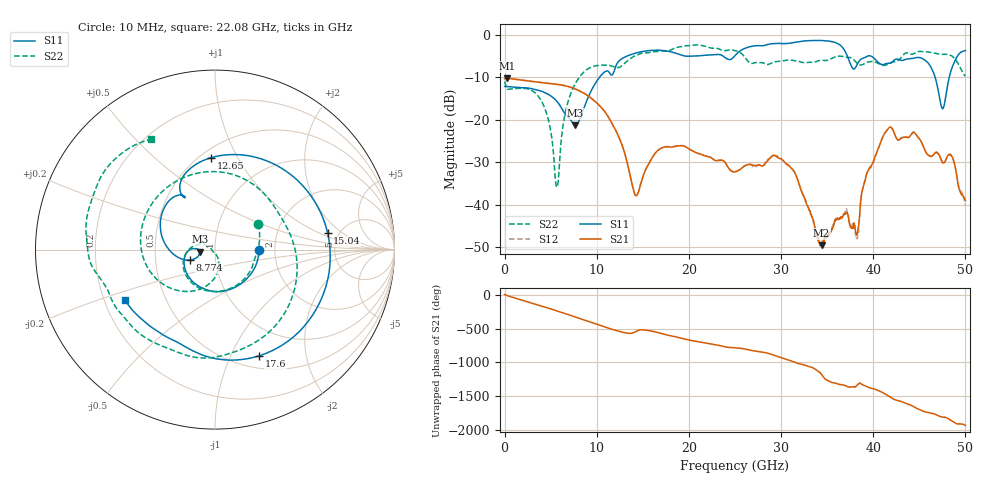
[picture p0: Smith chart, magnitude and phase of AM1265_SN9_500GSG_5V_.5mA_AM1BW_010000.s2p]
!Keysight Technologies,N5245B,MY58422270,A.16.20.02
!Date: Thursday, March 05, 2026 00:52:19
!Correction: S11(C  2-Port  )
!S21(C  2-Port  )
!S12(C  2-Port  )
!S22(C  2-Port  )
!S2P File: Measurements: S11, S21, S12, S22:
# Hz S  dB  R 50
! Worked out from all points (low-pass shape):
!   3201 points, 10 MHz to 50 GHz, reference 50 ohm
!   highest |S21| = -10.31 dB at 275.6 MHz (marker M1); lowest = -49.5 dB at 34.39 GHz (marker M2)
!   |S21| within 3 dB of the highest: start of sweep to 8.201 GHz
!   lowest |S11| = -21.3 dB at 7.68 GHz (marker M3), VSWR 1.19, Z = 42.1 - j1.01 ohm
!   |S11| at or under -10 dB: start of sweep to 10.32 GHz; 46.71 GHz to 48.25 GHz (1.541 GHz wide, 3.25 % of centre)
!   |S22| runs from -35.9 to -2.4 dB; largest |S21 - S12| = 0.0072
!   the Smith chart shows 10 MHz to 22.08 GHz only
!   S11 on the Smith chart (normalised r, x): 10 MHz: 1.65, -0.00; 8.774 GHz: 0.75, -0.09; 12.65 GHz: 0.57, +0.79; 15.04 GHz: 4.05, +1.27; 17.6 GHz: 0.64, -1.29; 22.08 GHz: 0.29, -0.24
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1e7  -12.20 -0.2  -10.37 4.3  -10.36 4.2  -11.05 30.8
2.755719e8  -12.23 -9.7  -10.31 -10.9  -10.29 -10.9  -12.81 -10.1
4.040444e9  -13.35 -128.9  -11.29 -167.0  -11.28 -167.0  -15.77 -172.9
5.680741e9  -15.69 -171.2  -11.70 122.7  -11.69 122.8  -35.87 -140.7
7.680341e9  -21.29 -172.1  -12.78 31.1  -12.78 31.2  -11.55 -119.0
8.352081e9  -18.86 -156.1  -13.47 -0.2  -13.46 -0.2  -9.40 -143.1
8.773872e9  -16.38 -157.5  -14.00 -19.9  -13.98 -19.9  -8.49 -158.6
1.110153e10  -8.55 132.4  -18.81 -127.1  -18.80 -127.1  -7.20 100.4
1.26481e10  -5.80 92.3  -25.39 171.4  -25.38 171.6  -7.46 13.9
1.503824e10  -3.95 8.5  -33.21 -158.7  -33.23 -159.1  -4.30 -99.9
1.667854e10  -3.67 -42.0  -27.16 158.7  -27.14 158.9  -4.00 -142.6
1.760023e10  -3.86 -67.5  -26.39 125.9  -26.31 126.0  -3.89 -159.7
2.208371e10  -4.81 -150.7  -28.70 -1.8  -28.65 -1.3  -2.96 120.0
2.5005e10  -4.96 175.5  -32.28 -64.2  -32.20 -63.7  -3.76 70.3
2.95041e10  -2.08 96.8  -28.66 172.5  -28.46 171.9  -6.35 -17.7
3.334708e10  -1.40 35.7  -42.85 3.7  -42.78 -0.9  -6.53 -132.1
3.439375e10  -1.40 17.4  -49.52 -101.0  -49.21 27.7  -6.06 -155.5
3.825235e10  -7.08 -22.0  -46.97 99.9  -48.01 106.5  -6.75 132.7
4.167354e10  -6.76 -54.5  -21.97 -58.8  -21.97 -58.7  -6.88 112.5
4.51416e10  -5.46 -100.8  -24.91 90.7  -24.90 91.1  -3.97 74.4
4.771921e10  -16.39 67.0  -30.11 -13.9  -30.17 -15.0  -4.62 40.5
5e10  -3.75 -70.7  -38.97 -135.6  -39.96 -131.5  -9.81 8.0
